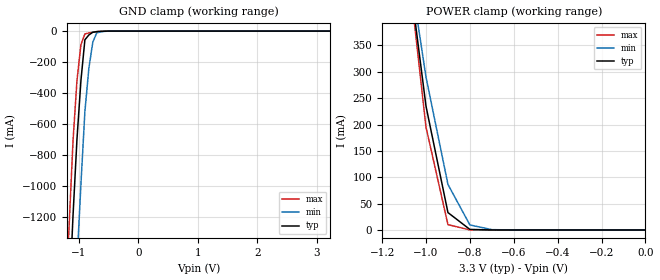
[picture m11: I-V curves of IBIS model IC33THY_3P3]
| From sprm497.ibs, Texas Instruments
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|   Model Cell IC33THY_3P3
|IC33THY_3P3
[Model]   IC33THY_3P3
Model_type   Input
Polarity   Non-Inverting
Vinl =  0.8V
Vinh =  2V
C_comp   0.8695239p   0.8584917p   0.8767304p
[Model Spec]
Vinl   0.8V   0.8V   0.8V
Vinh   2V   2V   2V
[Temperature Range]   25   125   -40
[Voltage Range]   3.3   2.97   3.465
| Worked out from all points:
|   GND clamp passes 1 mA (typ) near -0.58 V on its own axis
|   POWER clamp passes 1 mA (typ) near -0.80 V on its own axis
[POWER_clamp]
|   voltage   I(typ)   I(min)   I(max)
-3.3V     9.572A     8.115A     10.87A
-1.067V   452.1mA    472.8mA    444.6mA
-1.033V   343.5mA    381.5mA    319.8mA
-1V       234.9mA    290.2mA    195mA
-900mV    33.01mA    86.46mA    10.14mA
-800mV    1.012mA    9.543mA    89.45uA
-700mV    23.28uA    605.6uA    712.1nA
0V        217.5pA    10.6nA     11.51pA
[GND_clamp]
|   voltage   I(typ)   I(min)   I(max)
-3.3V     -22.43A    -23.21A    -22A
-1.233V   -2.35A     -3.221A    -1.845A
-1.167V   -1.763A    -2.627A    -1.266A
-1.1V     -1.191A    -2.042A    -709.2mA
-1.033V   -696.7mA   -1.494A    -318mA
-966.7mV  -318.5mA   -986.5mA   -87.77mA
-900mV    -56.12mA   -518.4mA   -18.69mA
-833.3mV  -25.12mA   -240.3mA   -12.29mA
-766.7mV  -7.66mA    -71.21mA   -7.13mA
-700mV    -3.747mA   -11.19mA   -3.213mA
-433.3mV  -54.28uA   -212.3uA   -16.6uA
3.233V    204.2pA    18.61nA    7.843pA
